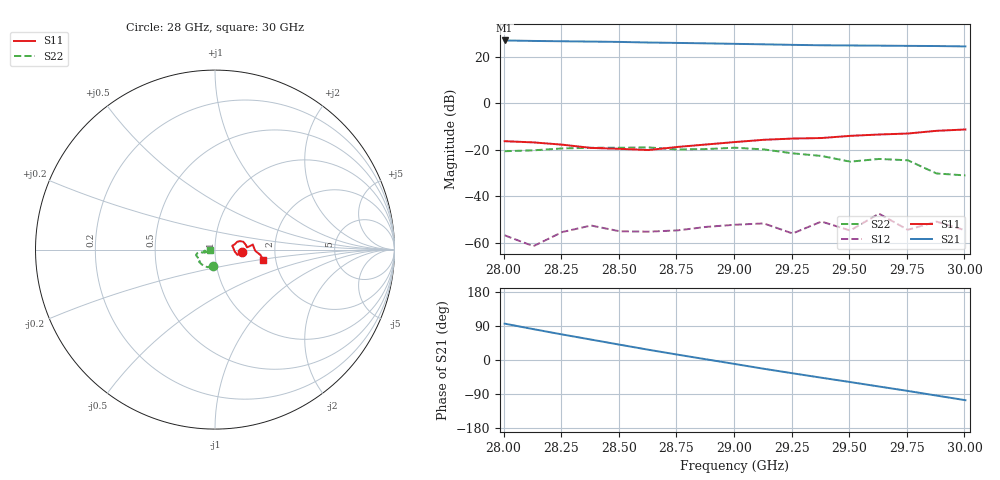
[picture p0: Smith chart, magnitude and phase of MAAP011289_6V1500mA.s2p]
!Keysight	"Technologies,N5247A,US51170177,A.10.64.09"
!Date:	"Friday,"	January	"04,"	2019	14:13:22
!Correction:	S11(Full	2	"Port(1,2))"
!S21(Full	2	"Port(1,2))"
!S12(Full	2	"Port(1,2))"
!S22(Full	2	"Port(1,2))"
!S2P	File:	Measurements:	"S11,"	"S21,"	"S12,"	S22:
# GHZ S DB R 50
!Freq DBS11 AngS11 DBS21 AngS21 DBS12 AngS12 DBS22 AngS22
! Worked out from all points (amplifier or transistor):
!   17 points, 28 GHz to 30 GHz, reference 50 ohm
!   highest |S21| = 27.0 dB at 28 GHz (marker M1)
!   |S21| within 3 dB of that: start of sweep to end of sweep
!   unconditionally stable (mu >= 1): start of sweep to end of sweep
!   at 28.25 GHz: K = 13.32, MAG = 26.8 dB, |S12| = -55.4 dB
!   at 29 GHz: K = 10.48, MAG = 25.7 dB, |S12| = -52.2 dB
!   at 30 GHz: K = 15.01, MAG = 24.8 dB, |S12| = -54.7 dB
28.0044  -16.32 -5.8  26.99 96.0  -56.79 155.7  -20.63 -97.8
28.12937  -16.84 -6.0  26.78 81.4  -61.46 35.5  -20.25 -106.0
28.25435  -17.81 -13.4  26.65 67.4  -55.38 -62.1  -19.43 -113.2
28.37933  -19.21 -5.1  26.51 53.9  -52.58 134.8  -19.16 -126.5
28.5043  -19.61 1.3  26.36 40.4  -55.06 45.3  -19.13 -133.4
28.62927  -20.12 12.8  26.10 27.0  -55.21 -103.6  -19.00 -142.6
28.75425  -18.80 15.1  25.93 14.2  -54.68 3.1  -19.87 -143.0
28.87923  -17.74 19.3  25.75 1.8  -53.17 -0.7  -19.71 -149.9
29.0042  -16.69 18.9  25.53 -10.6  -52.25 -106.8  -19.13 -163.8
29.12918  -15.72 15.4  25.33 -23.1  -51.68 -95.7  -19.86 -168.2
29.25415  -15.19 8.7  25.10 -35.0  -56.00 -55.9  -21.53 -171.0
29.37912  -14.96 4.1  24.92 -46.7  -50.88 -9.8  -22.65 -167.4
29.5041  -14.03 6.1  24.84 -58.2  -54.72 149.1  -25.12 -164.3
29.62908  -13.44 7.7  24.76 -69.9  -47.47 -82.4  -23.96 175.2
29.75405  -13.02 -1.5  24.66 -81.6  -54.42 18.3  -24.53 -164.9
29.87902  -11.86 -6.8  24.59 -93.9  -50.90 -175.8  -30.20 -170.7
30.004  -11.28 -12.0  24.44 -106.1  -54.65 -178.0  -31.04 -172.0
